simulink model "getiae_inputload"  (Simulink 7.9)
settings: Solver=ode23tb  StartTime=0.0  StopTime=400  RelTol=1e-6
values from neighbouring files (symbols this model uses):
  design = []    [sword.m]
libraries: simulink x2, cstextras x1

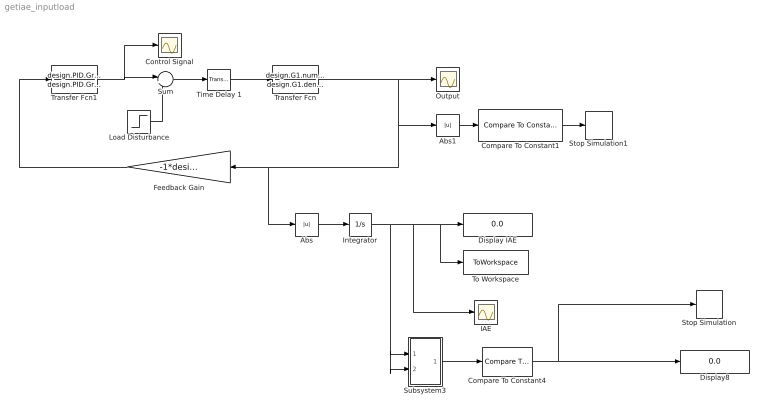
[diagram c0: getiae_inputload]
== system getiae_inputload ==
  Abs : Abs
  Abs1 : Abs
  Compare To Constant1 : simulink/Logic and Bit Operations/Compare To Constant  relop=>  const=5e12  OutDataTypeStr=boolean  ZeroCross=off
  Compare To Constant4 : simulink/Logic and Bit Operations/Compare To Constant  relop=<=  const=0.001  OutDataTypeStr=boolean  ZeroCross=off
  Control Signal : Scope
  Display IAE : Display
  Display8 : Display
  Feedback Gain : Gain  Gain=-1*design.sim.sgn
  IAE : Scope
  Integrator : Integrator
  Load Disturbance : Step  Time=0  SampleTime=0
  Output : Scope
  Stop Simulation : Stop
  Stop Simulation1 : Stop
  Subsystem3 : Subsystem
  Sum : Sum  Inputs=|++
  Time Delay 1 : cstextras/Transport Delay (masked)  Tag=InputDelayBlock  Td=design.sim.L1  u0=0  bufsize=100000
  To Workspace : ToWorkspace  VariableName=IAE_val  SampleTime=-1
  Transfer Fcn : TransferFcn  Numerator=design.G1.num{1}  Denominator=design.G1.den{1}
  Transfer Fcn1 : TransferFcn  Numerator=design.PID.Gr.num{1}  Denominator=design.PID.Gr.den{1}
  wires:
  Transfer Fcn1/1 -> Control Signal/1, Sum/1
  Time Delay 1/1 -> Transfer Fcn/1
  Feedback Gain/1 -> Transfer Fcn1/1
  Integrator/1 -> To Workspace/1, Display IAE/1, IAE/1, Subsystem3/1(In1), Subsystem3/2(In2)
  Subsystem3/1(Out1) -> Compare To Constant4/1
  Compare To Constant4/1 -> Display8/1, Stop Simulation/1
  Abs/1 -> Integrator/1
  Abs1/1 -> Compare To Constant1/1
  Compare To Constant1/1 -> Stop Simulation1/1
  Load Disturbance/1 -> Sum/2
  Sum/1 -> Time Delay 1/1
  Transfer Fcn/1 -> Output/1, Feedback Gain/1, Abs/1, Abs1/1

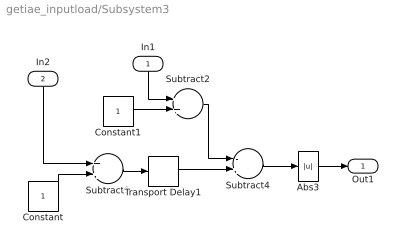
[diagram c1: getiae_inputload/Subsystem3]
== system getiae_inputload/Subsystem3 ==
  In1 : Inport
  In2 : Inport  Port=2
  Abs3 : Abs  ZeroCross=off
  Constant : Constant
  Constant1 : Constant
  Subtract1 : Sum
  Subtract2 : Sum
  Subtract4 : Sum  Inputs=-+
  Transport Delay1 : TransportDelay  DelayTime=50  BufferSize=100000
  Out1 : Outport
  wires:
  Abs3/1 -> Out1/1
  Subtract4/1 -> Abs3/1
  Transport Delay1/1 -> Subtract4/2
  Constant/1 -> Subtract1/2
  In2/1 -> Subtract1/1
  Subtract1/1 -> Transport Delay1/1
  Constant1/1 -> Subtract2/2
  Subtract2/1 -> Subtract4/1
  In1/1 -> Subtract2/1
